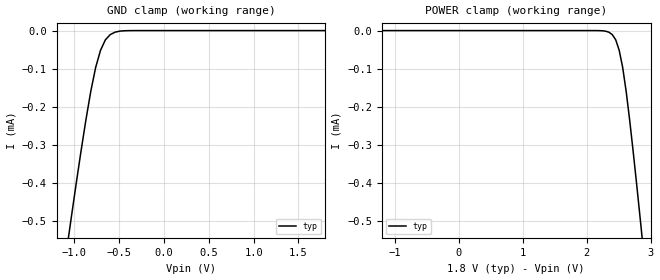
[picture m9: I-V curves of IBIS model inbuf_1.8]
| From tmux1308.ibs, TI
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| inbuf_1.8
[Model]   inbuf_1.8
Model_type   Input
Vinl = 0.6
Vinh = 0.95
|   typ   min   max
C_comp   2.533030e-14   NA   NA
[Voltage Range]   1.8   NA   NA
[Temperature Range]   27   NA   NA
[Power Clamp Reference]   1.8   NA   NA
[GND Clamp Reference]   0   NA   NA
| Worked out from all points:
|   GND clamp passes 1 mA (typ) near -1.33 V on its own axis
[GND Clamp]
|   Voltage   I(typ)   I(min)   I(max)
-3.6V     -5.119mA   NA         NA
-1.091V   -582.7uA   NA         NA
-1.036V   -492.1uA   NA         NA
-872.7mV  -235.2uA   NA         NA
-818.2mV  -160uA     NA         NA
-763.6mV  -97.04uA   NA         NA
-709.1mV  -51.81uA   NA         NA
-654.5mV  -24.23uA   NA         NA
-600mV    -10.45uA   NA         NA
-490.9mV  -1.356uA   NA         NA
-381.8mV  -104nA     NA         NA
1.8V      26.17pA    NA         NA
[POWER Clamp]
|   Voltage   I(typ)   I(min)   I(max)
-1.8V     173.9pA    NA         NA
2.127V    -23.87nA   NA         NA
2.345V    -4.04uA    NA         NA
2.4V      -10.45uA   NA         NA
2.455V    -24.23uA   NA         NA
2.509V    -51.81uA   NA         NA
2.564V    -97.04uA   NA         NA
2.618V    -160uA     NA         NA
2.673V    -235.2uA   NA         NA
2.836V    -492.1uA   NA         NA
2.891V    -582.7uA   NA         NA
3.6V      -1.827mA   NA         NA
